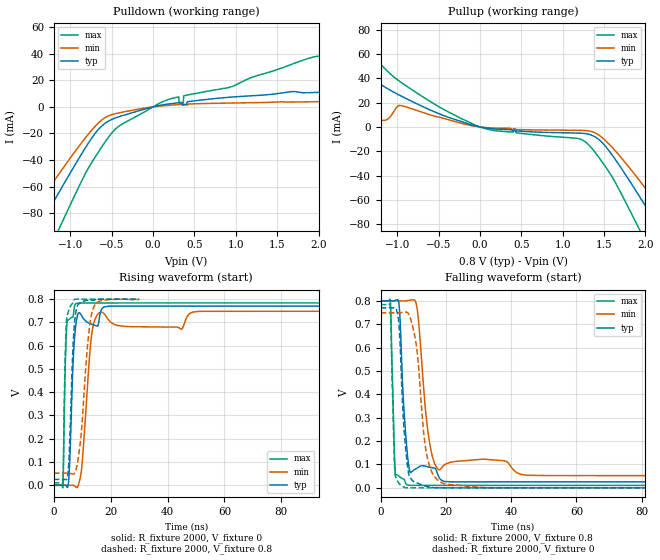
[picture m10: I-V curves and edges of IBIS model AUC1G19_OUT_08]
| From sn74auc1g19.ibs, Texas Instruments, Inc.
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[Model]   AUC1G19_OUT_08
Model_type  Output
Vref =   0
Rref =   2000
Cref =   15p
Vmeas =   0.4
| variable   typ   min   max
C_comp   5.26pF   2.57pF   7.93pF
| C_pullup   5.26pF   2.57pF   7.93pF
| C_pulldown   5.26pF   2.57pF   7.93pF
[Temperature Range]   40   100   -40
| Ambient temperature   25   85   -40
[Voltage range]   0.8   0.8   0.8
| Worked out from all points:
|   slope of the pulldown table from 0 to 0.12 V, typ, clamps not added: 77.1 ohm
|   slope of the pullup table from 0 to 0.12 V, typ, clamps not added: 93 ohm
|   rising waveform, R_fixture 2000, V_fixture 0: 20-80 % time 1.43ns typ, 2.57ns min, 821ps max; typ from 0 V to 0.77 V
|   falling waveform, R_fixture 2000, V_fixture 0.8: 20-80 % time 1.78ns typ, 2.91ns min, 869ps max; typ from 0.8 V to 0.025 V
|   rising waveform, R_fixture 2000, V_fixture 0.8: 20-80 % time 1.42ns typ, 2.77ns min, 770ps max; typ from 0.025 V to 0.8 V
|   falling waveform, R_fixture 2000, V_fixture 0: 20-80 % time 1.8ns typ, 2.98ns min, 865ps max; typ from 0.77 V to 0 V
[Pulldown]
| AUC1G19_OUT_08
|   Voltage   I(typ)   I(min)   I(max)
-3.6V     -335.8mA   -281.6mA   -413.5mA
-1.635V   -118.7mA   -95.5mA    -157.6mA
-1.375V   -90.1mA    -71.65mA   -123.3mA
-1.155V   -66.15mA   -51.9mA    -94.08mA
-630mV    -14.97mA   -10.4mA    -31.03mA
-430mV    -7.788mA   -4.787mA   -15.34mA
-90mV     -1.494mA   -794.3uA   -3.292mA
210mV     2.329mA    1.254mA    6.027mA
365mV     1.692mA    1.285mA    2.781mA
1.97V     10.82mA    3.859mA    37.81mA
2.35V     11.7mA     4.186mA    33.41mA
7.2V      23.85mA    8.894mA    59.34mA
[Pullup]
| AUC1G19_OUT_08
|   Voltage   I(typ)   I(min)   I(max)
-3.6V     79.23mA    9.066mA    183.6mA
-3.08V    77.72mA    9.395mA    160.6mA
-1.585V   27.6mA     10.91mA    82.19mA
-1.305V   38.33mA    6.636mA    59.52mA
-1.13V    31.97mA    5.798mA    46.56mA
-975mV    26.17mA    17.65mA    37.64mA
-235mV    4.613mA    3.12mA     7.149mA
1.36V     -7.061mA   -3.985mA   -18.17mA
1.87V     -50.82mA   -38.91mA   -76.44mA
2.115V    -77.26mA   -60.45mA   -109.4mA
2.4V      -108.6mA   -86.34mA   -147.6mA
7.2V      -641.3mA   -545mA     -778.8mA
[Ramp]
| AUC1G19_OUT_08
| variable   typ   min   max
dV/dt_r   0.47/1.44E-09   0.46/2.59E-09   0.48/8.27E-10
dV/dt_f   0.47/1.78E-09   0.45/2.91E-09   0.48/8.76E-10
R_load = 2000
[Rising Waveform]
| AUC1G19_OUT_08
R_fixture =   2000
C_fixture =   0
L_fixture =   0
V_fixture =   0
V_fixture_min = 0
V_fixture_max = 0
|   Time   V(typ)   V(min)   V(max)
0s        8.052nV    45.46nV    527.4pV
3.18ns    82.01uV    -7.373uV   -6.866mV
4.235ns   -579.1uV   -15.53uV   603mV
5.145ns   10.54mV    281.7uV    710.9mV
6.875ns   551.6mV    -304.9uV   731.9mV
8.005ns   712.2mV    -9.193mV   781.6mV
9.835ns   727.4mV    78.9mV     783.5mV
13.34ns   692mV      650.2mV    783.7mV
16.42ns   744.7mV    743.6mV    783.7mV
210ns     770mV      748.6mV    783.8mV
[Falling Waveform]
| AUC1G19_OUT_08
R_fixture =   2000
C_fixture =   0
L_fixture =   0
V_fixture =   0.8
V_fixture_min = 0.8
V_fixture_max = 0.8
|   Time   V(typ)   V(min)   V(max)
0s        800mV      800mV      800mV
2.945ns   800mV      800mV      802.4mV
4.34ns    800.8mV    800mV      95.52mV
5.505ns   795.9mV    799.8mV    51.61mV
8.055ns   162.2mV    800.5mV    13.16mV
9.055ns   65.77mV    802.6mV    10.99mV
11.05ns   83.72mV    777.2mV    10.68mV
14.5ns    89.64mV    239mV      10.64mV
17.8ns    46.88mV    76.9mV     10.63mV
110ns     25.47mV    52.27mV    10.6mV
[Rising Waveform]
| AUC1G19_OUT_08
R_fixture =   2000
C_fixture =   0
L_fixture =   0
V_fixture =   0.8
V_fixture_min = 0.8
V_fixture_max = 0.8
|   Time   V(typ)   V(min)   V(max)
0s        25.46mV    52.25mV    10.6mV
3.14ns    25.53mV    52.24mV    9.747mV
4.31ns    23.82mV    52.32mV    671.6mV
5.155ns   79.73mV    52.15mV    748.4mV
5.735ns   242.9mV    51.14mV    767.3mV
6.94ns    639.8mV    48.4mV     792.6mV
8.375ns   773.2mV    98.28mV    799.6mV
12.21ns   795.7mV    644.7mV    799.9mV
13.87ns   794.3mV    760.6mV    799.9mV
29.99ns   800mV      798.7mV    800mV
[Falling Waveform]
| AUC1G19_OUT_08
R_fixture =   2000
C_fixture =   0
L_fixture =   0
V_fixture =   0
V_fixture_min = 0
V_fixture_max = 0
|   Time   V(typ)   V(min)   V(max)
0s        770mV      748.6mV    783.8mV
2.925ns   770mV      748.6mV    773.2mV
4.265ns   771.3mV    748.6mV    93.41mV
5.295ns   735.1mV    748.6mV    25.82mV
7.45ns    201.3mV    751.5mV    1.295mV
8.63ns    57.35mV    742.3mV    177.8uV
10.78ns   22.64mV    624.5mV    68.38uV
14.41ns   5.529mV    122mV      38.53uV
19.53ns   142.7uV    17.45mV    24uV
210ns     4.749uV    -674.9nV   2.092uV
